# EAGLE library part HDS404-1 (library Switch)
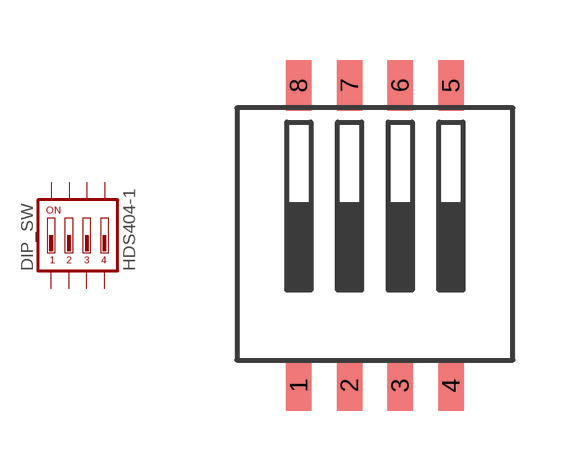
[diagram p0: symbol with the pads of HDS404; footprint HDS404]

Designator prefix DIP_SW

## HDS404-1  [HDS404]
1  1  pas
2  2  pas
3  3  pas
4  4  pas
5  5  pas
6  6  pas
7  7  pas
8  8  pas

## Footprint HDS404 (pad centres in mm)
smd 0.635 x 1.27: 1 -1.905,-3.785; 2 -0.635,-3.785; 3 0.635,-3.785; 4 1.905,-3.785; 5 1.905,3.715; 6 0.635,3.715; 7 -0.635,3.715; 8 -1.905,3.715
